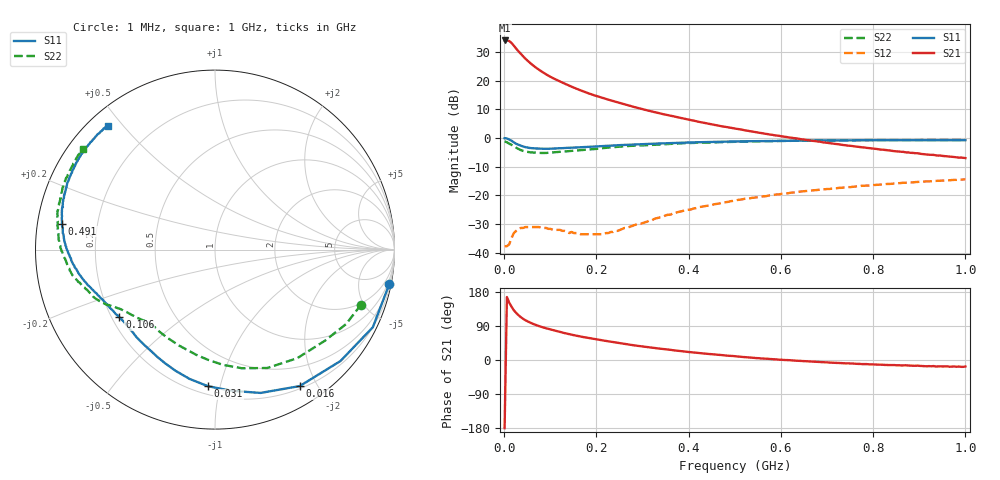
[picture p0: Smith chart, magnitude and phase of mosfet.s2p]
! RD16HHF1 S-parameters
! Ta=25deg. C, VDS=12.5V, IDS=500mA
! 7th Apr. 2003
# GHZ S MA R 50
!  Freq.  S11  S21  S12  S22
!  GHz  (mag)  (ang)  (mag)  (ang)  (mag)  (ang)  (mag)  (ang)
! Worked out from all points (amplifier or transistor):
!   201 points, 1 MHz to 1 GHz, reference 50 ohm
!   highest |S21| = 34.0 dB at 1 MHz (marker M1)
!   |S21| within 3 dB of that: start of sweep to 26.94 MHz
!   unconditionally stable (mu >= 1): 191.9 MHz to 230.6 MHz; 232.5 MHz to 237.3 MHz
!   at 166 MHz: K = 0.88, MSG = 25.1 dB, |S12| = -33.6 dB
!   at 501 MHz: K = 0.42, MSG = 12.5 dB, |S12| = -21.8 dB
!   at 1 GHz: K = 0.52, MSG = 3.7 dB, |S12| = -14.4 dB
!   S11 on the Smith chart (normalised r, x): 1 MHz: 1, -10; 16 MHz: 0.23, -1.78; 31 MHz: 0.25, -0.92; 106 MHz: 0.23, -0.30; 491 MHz: 0.07, +0.08; 1 GHz: 0.05, +0.46
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0.001  0.99 -11.2  50.03 180.2  0.013 60.6  0.87 -20.6
0.006  0.98 -26.2  50.03 166.2  0.013 60.6  0.84 -29.6
0.011  0.935 -41.6  48.87 151.3  0.014 62.6  0.796 -39.5
0.016  0.895 -58.2  45.24 140.7  0.018 56.8  0.759 -52.9
0.021  0.838 -72.3  40.6 131.3  0.022 47.7  0.721 -66.2
0.026  0.792 -83.4  36.15 124.3  0.024 39.9  0.678 -77.2
0.031  0.762 -93.0  32.44 118.4  0.026 34.8  0.643 -86.2
0.036  0.734 -101.2  29.32 113.1  0.027 31.3  0.615 -93.7
0.041  0.71 -108.1  26.53 108.8  0.027 28.4  0.595 -100.3
0.046  0.692 -113.5  24.09 105.0  0.028 27.0  0.58 -105.5
0.056  0.668 -122.3  20.39 98.9  0.028 21.4  0.563 -114.4
0.076  0.65 -134.5  15.36 89.2  0.028 17.6  0.548 -126.4
0.106  0.652 -144.7  11.02 78.8  0.025 17.9  0.559 -134.9
0.141  0.673 -152.6  8.151 68.3  0.022 22.4  0.59 -141.9
0.171  0.692 -157.1  6.509 60.7  0.021 30.1  0.615 -146.7
0.246  0.746 -166.1  4.174 45.2  0.024 60.7  0.702 -155.6
0.336  0.802 -175.4  2.703 30.3  0.041 78.7  0.769 -165.2
0.491  0.865 170.3  1.508 11.0  0.079 76.7  0.856 -179.6
0.501  0.867 169.5  1.456 9.9  0.081 76.0  0.86 179.5
0.671  0.903 155.5  0.887 -4.3  0.122 66.1  0.902 165.7
0.836  0.914 142.9  0.605 -13.3  0.158 55.1  0.918 153.9
1  0.914 130.8  0.446 -17.2  0.19 43.7  0.924 142.5
